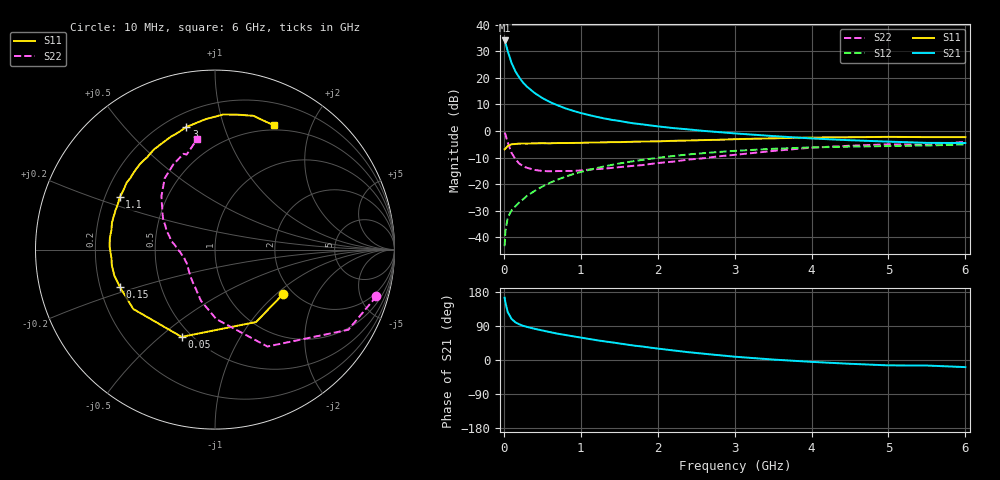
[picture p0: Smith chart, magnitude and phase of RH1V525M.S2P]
! SIEMENS Small Signal Semiconductors
! BFR106
! Si NPN RF Bipolar Junction Transistor in SOT23
! VCE = 1.5 V  IC = 25 mA
! Common Emitter S-Parameters:  August  1996
# GHz  S  MA  R  50
!  f  S11  S21  S12  S22
! GHz  MAG  ANG  MAG  ANG  MAG  ANG  MAG  ANG
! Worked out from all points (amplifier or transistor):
!   36 points, 10 MHz to 6 GHz, reference 50 ohm
!   highest |S21| = 34.1 dB at 10 MHz (marker M1)
!   |S21| within 3 dB of that: start of sweep to 40.81 MHz
!   unconditionally stable (mu >= 1): 309.1 MHz to 2.868 GHz; 4.712 GHz to end of sweep
!   at 250 MHz: K = 0.95, MSG = 22.0 dB, |S12| = -25.7 dB
!   at 1.4 GHz: K = 1.08, MAG = 6.8 dB, |S12| = -12.8 dB
!   at 6 GHz: K = 1.02, MAG = -0.5 dB, |S12| = -5.1 dB
!   S11 on the Smith chart (normalised r, x): 10 MHz: 1.79, -1.11; 50 MHz: 0.44, -0.59; 150 MHz: 0.28, -0.18; 1.1 GHz: 0.26, +0.24; 3 GHz: 0.28, +0.75; 6 GHz: 0.44, +1.49
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0.01  0.4533 -32.9  50.59 164.5  0.0068 78.2  0.9365 -16.1
0.02  0.464 -60.4  46.25 152.2  0.0128 70.1  0.8669 -31.0
0.05  0.5207 -110.9  31.99 126.7  0.0234 54.8  0.6138 -61.6
0.1  0.5629 -144.0  19.17 108.4  0.0321 51.6  0.3871 -89.0
0.15  0.5694 -158.5  13.27 99.5  0.0382 53.5  0.2954 -105.4
0.2  0.5795 -165.7  10.18 94.3  0.0453 56.6  0.2443 -115.8
0.25  0.5813 -171.3  8.156 90.2  0.0518 59.0  0.2169 -125.6
0.3  0.579 -175.1  6.842 87.4  0.06 61.9  0.2033 -132.0
0.4  0.5872 178.4  5.193 82.4  0.0745 63.8  0.1853 -142.9
0.5  0.5894 173.8  4.175 77.9  0.09 65.1  0.1768 -150.2
0.6  0.5873 169.2  3.505 73.6  0.1062 65.3  0.1746 -154.8
0.7  0.5934 165.3  3.036 69.4  0.1219 65.0  0.1761 -159.1
0.9  0.5959 158.5  2.401 62.5  0.154 63.4  0.177 -166.7
1.1  0.6059 151.2  2.007 55.7  0.1844 61.1  0.1873 -171.2
1.3  0.6117 145.3  1.73 49.4  0.2148 58.2  0.1954 -176.5
1.6  0.6233 137.1  1.457 40.7  0.2584 53.8  0.2155 177.1
2.2  0.6531 121.5  1.137 25.3  0.3383 44.1  0.2651 163.6
3  0.7015 103.1  0.902 8.7  0.423 30.9  0.3555 145.4
3.5  0.7286 94.1  0.803 1.2  0.4631 23.2  0.4214 135.1
4.5  0.7634 79.7  0.67 -10.0  0.5078 8.7  0.5281 116.1
5.5  0.767 68.5  0.598 -14.6  0.5328 0.0  0.5526 106.6
6  0.7662 64.7  0.594 -18.8  0.5579 -6.8  0.624 99.1
